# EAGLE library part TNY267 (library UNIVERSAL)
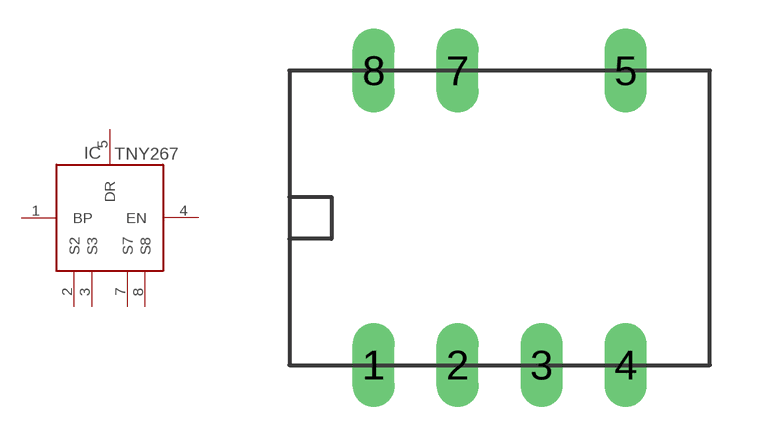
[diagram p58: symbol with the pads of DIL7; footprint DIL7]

Designator prefix IC

## TNY267 (IC: TNY267)  [DIL7]
1  BP
2  S2
3  S3
4  EN
5  DR
7  S7
8  S8

## Footprint DIL7 (pad centres in mm)
drill 0.61 pad 1.27 long: 1 2.54,0; 2 5.08,0; 3 7.62,0; 4 10.16,0; 5 10.16,8.89; 7 5.08,8.89; 8 2.54,8.89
